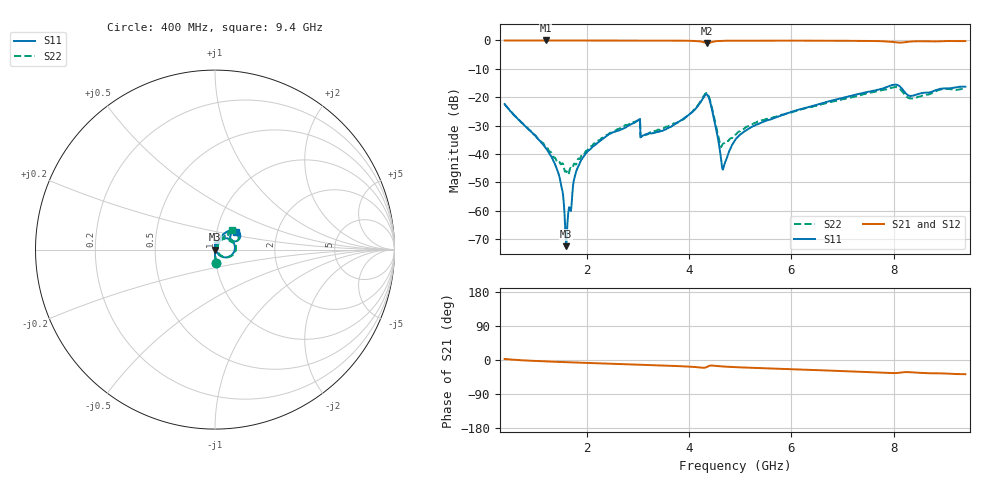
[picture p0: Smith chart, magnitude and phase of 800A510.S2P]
!  American Technical Ceramics  Date:  9/12/2007
!  One Norden Lane
!  Huntington Station,  NY.  11746-2102
!  Tel:  (631) 622-4700  Fax:  (631) 622-4748
!  Part Number  800A510  Mounting Orientation: Vertical
!  Description: Ultra Low ESR Microwave capacitors
!  Application: Coupling, Bypass, Tuning, DC Block
!  Filters, Matching
# GHZ S DB R 50
! Freq  |S11|  S11 Ph  |S21|  S21 Ph  |S12|  S12 Ph  |S22|  S22 Ph
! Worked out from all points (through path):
!   801 points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, 400 MHz to 9.4 GHz, reference 50 ohm
!   highest |S21| = -0.03 dB at 1.199 GHz (marker M1); lowest = -1.1 dB at 4.36 GHz (marker M2)
!   group delay of S21, straight-line fit = 11.8 ps
!   lowest |S11| = -72.4 dB at 1.604 GHz (marker M3), VSWR 1.00, Z = 50 + j0.00996 ohm
!   |S11| at or under -10 dB: start of sweep to end of sweep
!   |S22| runs from -47.2 to -16.4 dB; largest |S21 - S12| = 0.0018
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0.4  -22.41 -86.2  -0.05 2.8  -0.04 2.9  -22.45 -85.8
1.199  -37.78 -94.1  -0.03 -3.6  -0.03 -3.6  -37.48 -77.4
1.458  -47.13 -101.4  -0.04 -5.0  -0.03 -5.0  -42.49 -49.4
1.604  -72.41 155.4  -0.04 -5.7  -0.03 -5.8  -46.04 -23.6
1.649  -59.78 80.7  -0.04 -6.0  -0.03 -6.0  -47.19 -3.2
1.784  -46.99 108.2  -0.05 -6.6  -0.04 -6.6  -43.66 21.9
1.908  -41.80 95.8  -0.05 -7.2  -0.04 -7.2  -40.28 40.0
2.391  -33.66 89.0  -0.06 -9.5  -0.05 -9.5  -33.29 55.6
2.999  -28.31 88.3  -0.08 -12.3  -0.07 -12.3  -28.14 60.2
3.1  -33.52 82.7  -0.07 -12.7  -0.06 -12.7  -33.76 53.1
3.404  -32.16 77.6  -0.09 -14.1  -0.08 -14.1  -31.42 55.9
3.865  -27.89 76.8  -0.12 -16.6  -0.11 -16.6  -28.00 61.3
4.36  -19.18 -0.5  -1.08 -17.8  -1.07 -17.8  -18.71 -1.6
4.45  -24.40 -43.5  -0.58 -14.6  -0.57 -14.6  -23.79 -39.8
4.596  -37.68 -52.7  -0.21 -16.5  -0.21 -16.5  -35.50 -30.1
4.664  -45.48 2.5  -0.17 -17.0  -0.17 -17.0  -36.39 9.7
4.9  -35.15 71.3  -0.11 -18.8  -0.10 -18.9  -33.21 47.3
5.271  -30.08 72.0  -0.10 -20.9  -0.10 -20.9  -29.11 59.0
6.408  -23.11 66.4  -0.12 -26.3  -0.12 -26.3  -23.40 58.2
7.904  -16.08 46.2  -0.42 -34.3  -0.42 -34.4  -17.03 41.3
8.343  -19.53 34.3  -0.40 -32.4  -0.40 -32.5  -20.44 33.2
9.4  -16.28 40.6  -0.25 -37.5  -0.26 -37.6  -16.82 49.9
